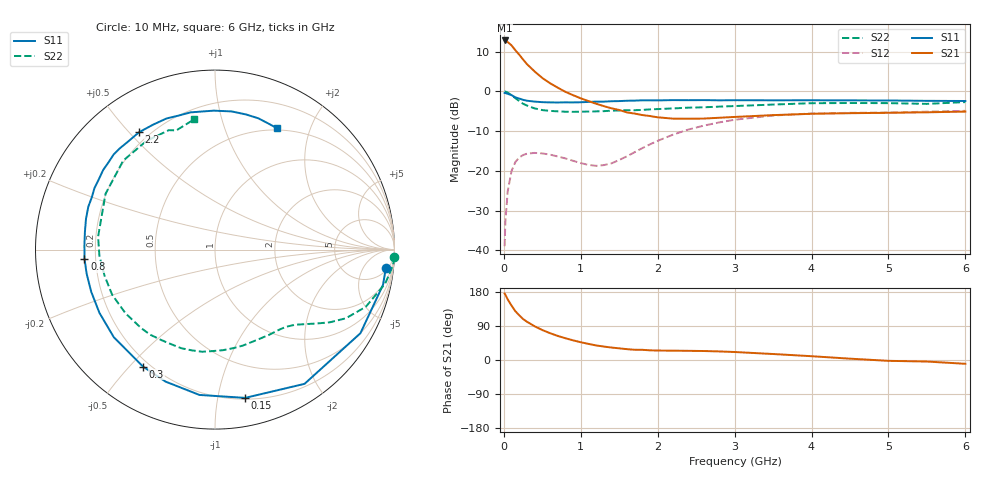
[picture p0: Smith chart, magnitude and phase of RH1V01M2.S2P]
! SIEMENS Small Signal Semiconductors
! BFR106
! Si NPN RF Bipolar Junction Transistor in SOT23
! VCE = 1 V  IC = 1.2 mA
! Common Emitter S-Parameters:  August  1996
# GHz  S  MA  R  50
!  f  S11  S21  S12  S22
! GHz  MAG  ANG  MAG  ANG  MAG  ANG  MAG  ANG
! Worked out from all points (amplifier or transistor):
!   36 points, 10 MHz to 6 GHz, reference 50 ohm
!   highest |S21| = 12.8 dB at 10 MHz (marker M1)
!   |S21| within 3 dB of that: start of sweep to 174.1 MHz
!   unconditionally stable (mu >= 1): 818.6 MHz to end of sweep
!   at 250 MHz: K = 0.30, MSG = 12.0 dB, |S12| = -16.0 dB
!   at 1.4 GHz: K = 1.52, MAG = 2.7 dB, |S12| = -18.1 dB
!   at 6 GHz: K = 1.02, MAG = -1.0 dB, |S12| = -4.9 dB
!   S11 on the Smith chart (normalised r, x): 10 MHz: 6, -16; 150 MHz: 0.21, -1.20; 300 MHz: 0.17, -0.55; 800 MHz: 0.16, -0.03; 2.2 GHz: 0.16, +0.53; 6 GHz: 0.48, +1.52
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0.01  0.9576 -6.2  4.387 175.3  0.0113 87.8  0.9992 -2.4
0.02  0.9564 -11.9  4.342 172.3  0.0227 81.8  0.9969 -4.8
0.05  0.9346 -29.9  4.188 160.0  0.0552 72.6  0.9672 -11.3
0.1  0.8991 -56.3  3.806 143.7  0.0998 58.4  0.8984 -20.8
0.15  0.843 -78.5  3.305 128.7  0.1295 46.1  0.8233 -27.7
0.2  0.8144 -96.1  2.905 118.0  0.1477 37.7  0.7579 -32.3
0.25  0.7854 -110.5  2.526 108.1  0.1585 30.4  0.7004 -36.0
0.3  0.7652 -121.6  2.213 101.0  0.1649 25.8  0.6656 -38.5
0.4  0.7458 -139.1  1.786 89.0  0.1686 18.2  0.6123 -43.1
0.5  0.734 -151.3  1.479 79.1  0.1662 13.4  0.5834 -47.6
0.6  0.7286 -161.2  1.271 70.8  0.1604 10.8  0.5697 -52.2
0.8  0.7289 -176.0  0.99 57.4  0.1438 9.5  0.5563 -62.6
1.1  0.7389 166.6  0.757 42.5  0.1191 20.0  0.5586 -79.5
1.3  0.7456 157.0  0.654 35.5  0.1184 34.6  0.5654 -91.2
1.6  0.7648 144.6  0.545 28.6  0.1527 53.1  0.5807 -109.0
2.2  0.7788 122.9  0.455 24.6  0.2864 55.5  0.612 -144.5
2.8  0.7737 105.2  0.467 22.6  0.408 42.5  0.645 -177.0
3.5  0.7742 90.5  0.504 15.8  0.4981 26.3  0.6845 153.0
4.5  0.7725 77.0  0.533 3.5  0.5386 7.8  0.7157 122.3
5  0.7703 71.7  0.539 -2.2  0.5429 1.0  0.7134 111.1
5.5  0.7626 66.9  0.547 -4.1  0.5571 -2.3  0.6982 108.0
6  0.7592 63.1  0.558 -10.0  0.5705 -9.1  0.7354 99.0
